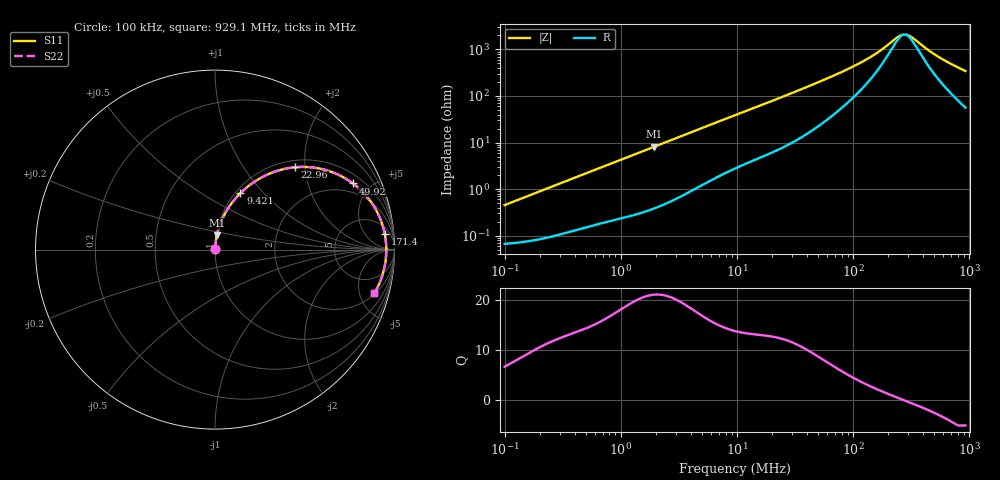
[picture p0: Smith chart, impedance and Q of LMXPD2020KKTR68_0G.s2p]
! LMXPD2020KKTR68_0G  S-PARAMETER MODEL  ( General Type )
! Model Generated by TAIYO YUDEN Corporation (https://www.yuden.co.jp/en/)
! Version 1.0
! TAIYO YUDEN Control No. 191023NI43SB-FBB
! Copyright(c) 2019 TAIYO YUDEN CO.,LTD. All Rights Reserved.
! Product Description (link to TY-COMPAS)
! https://ds.yuden.co.jp/TYCOMPAS/or/detail?pn=LMXPD2020KKTR68N0G&u=M
! Products Name : Inductors
! Characteristics :
!  Inductance : 0.68 uH , SRF(min) : -Hz , DC Resistance(max) : 0.072 Ohm
!  Rated Current : Saturation :1850 mA , Temp Rise : 1850 mA (40 degC)
!  Case Size : 2.0 x 2.0 / 0.079 x 0.079 [mm/inch] , Thickness : 1 / 0.039 [mm/inch]
!  (Conditions: Temperature = 25 degC , DC Bias Current/Voltage = 0A / 0V)
! External Node Assignments :
!  1  o---GGG---o  2
! GND o---------o GND
! Frequency Range : 0.1MHz  -  929.055398MHz  [ 402 STEP ]
# MHz S RI R 50
! Freq[MHz].  S11 Real  S11 Imag  S21 Real  S21 Imag  S12 Real  S12 Imag  S22 Real  S22 Imag
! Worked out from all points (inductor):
!   401 points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, 100 kHz to 929.1 MHz, reference 50 ohm
!   read as one part in series: L = 713 nH near 104.7 kHz
!   highest Q = 21.2 at 1.948 MHz (marker M1), where L = 667 nH
!   self-resonance near 278.3 MHz
!   S11 on the Smith chart (normalised r, x): 100 kHz: 1.00, +0.01; 9.421 MHz: 1.05, +0.75; 22.96 MHz: 1.14, +1.78; 49.92 MHz: 1.44, +3.89; 171.4 MHz: 9, +17; 929.1 MHz: 2.13, -6.78
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0.1  0.000686 0.00448  0.9993 -0.00448  0.9993 -0.00448  0.000686 0.00448
0.462005  0.00183 0.0201  0.9982 -0.0201  0.9982 -0.0201  0.00183 0.0201
1.94811  0.0104 0.0805  0.9896 -0.0805  0.9896 -0.0805  0.0104 0.0805
2.134489  0.012 0.0879  0.988 -0.0879  0.988 -0.0879  0.012 0.0879
4.969787  0.0505 0.1915  0.9495 -0.1915  0.9495 -0.1915  0.0505 0.1915
9.42108  0.1415 0.3145  0.8585 -0.3145  0.8585 -0.3145  0.1415 0.3145
9.638752  0.1465 0.3194  0.8535 -0.3194  0.8535 -0.3194  0.1465 0.3194
14.54061  0.2615 0.4032  0.7385 -0.4032  0.7385 -0.4032  0.2615 0.4032
22.96068  0.4468 0.4588  0.5532 -0.4588  0.5532 -0.4588  0.4468 0.4588
31.61304  0.5923 0.4494  0.4077 -0.4494  0.4077 -0.4494  0.5923 0.4494
44.53155  0.7305 0.3943  0.2695 -0.3943  0.2695 -0.3943  0.7305 0.3943
49.91928  0.7686 0.3687  0.2314 -0.3687  0.2314 -0.3687  0.7686 0.3687
70.31854  0.8558 0.2838  0.1442 -0.2838  0.1442 -0.2838  0.8558 0.2838
101.3425  0.9107 0.1948  0.0893 -0.1948  0.0893 -0.1948  0.9107 0.1948
133.3008  0.9338 0.1351  0.0662 -0.1351  0.0662 -0.1351  0.9338 0.1351
171.3775  0.9461 0.0859  0.0539 -0.0859  0.0539 -0.0859  0.9461 0.0859
205.7381  0.9512 0.0525  0.0488 -0.0525  0.0488 -0.0525  0.9512 0.0525
258.5329  0.9541 0.0127  0.0459 -0.0127  0.0459 -0.0127  0.9541 0.0127
296.508  0.9543 -0.0109  0.0457 0.0109  0.0457 0.0109  0.9543 -0.0109
536.9812  0.9394 -0.1195  0.0606 0.1195  0.0606 0.1195  0.9394 -0.1195
722.6375  0.9181 -0.183  0.0819 0.183  0.0819 0.183  0.9181 -0.183
929.0554  0.888 -0.2432  0.112 0.2432  0.112 0.2432  0.888 -0.2432
